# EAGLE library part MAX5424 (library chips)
Variable POT 256 Tap
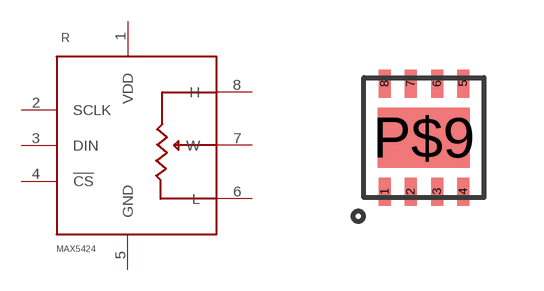
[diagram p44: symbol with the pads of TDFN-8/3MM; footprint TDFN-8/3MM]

Designator prefix R

## MAX5424  [TDFN-8/3MM]
1  VDD
2  SCLK
3  DIN
4  !CS
5  GND
6  L
7  W
8  H

## Footprint TDFN-8/3MM (pad centres in mm)
smd 0.3 x 0.7: 1 -0.98,-1.35; 2 -0.33,-1.35; 3 0.33,-1.35; 4 0.98,-1.35; 5 0.98,1.35; 6 0.33,1.35; 7 -0.33,1.35; 8 -0.98,1.35
smd 2.3 x 1.5: P$9 0,0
